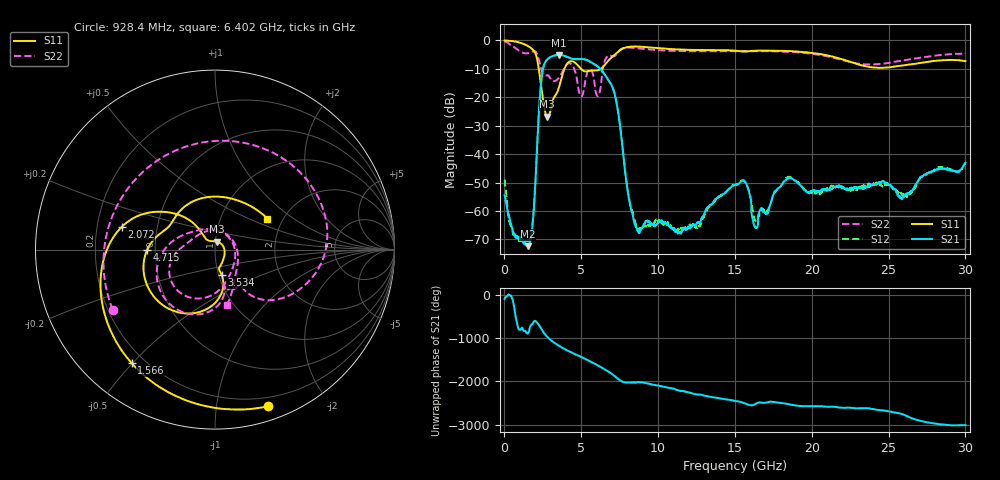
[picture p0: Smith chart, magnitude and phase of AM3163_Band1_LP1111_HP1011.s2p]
!Agilent Technologies,E8364B,MY43040894,A.07.50.67
!Agilent E8364B: A.07.50.67
!Date: Thursday, August 20, 2020 12:00:17
!Correction: S11(Full 2 Port(1,2))
!S21(Full 2 Port(1,2))
!S12(Full 2 Port(1,2))
!S22(Full 2 Port(1,2))
!S2P File: Measurements: S11, S21, S12, S22:
# Hz S  dB  R 50
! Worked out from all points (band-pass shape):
!   3201 points, 10 MHz to 30 GHz, reference 50 ohm
!   highest |S21| = -5.13 dB at 3.553 GHz (marker M1); lowest = -72.4 dB at 1.51 GHz (marker M2)
!   |S21| within 3 dB of the highest: 2.614 GHz to 5.778 GHz (3.164 GHz wide, 75.4 % of centre)
!   lowest |S11| = -26.9 dB at 2.775 GHz (marker M3), VSWR 1.09, Z = 50.7 + j4.51 ohm
!   |S11| at or under -10 dB: 2.233 GHz to 3.901 GHz (1.668 GHz wide, 54.4 % of centre); 4.978 GHz to 6.273 GHz (1.295 GHz wide, 23 % of centre)
!   |S22| runs from -19.8 to -0.3 dB; largest |S21 - S12| = 0.0055
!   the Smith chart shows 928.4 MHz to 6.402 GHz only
!   S11 on the Smith chart (normalised r, x): 928.4 MHz: 0.12, -1.39; 1.566 GHz: 0.15, -0.50; 2.072 GHz: 0.31, +0.11; 3.534 GHz: 1.03, -0.30; 4.715 GHz: 0.45, -0.00; 6.402 GHz: 1.67, +0.65
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1e7  -0.04 -4.9  -54.47 -93.1  -48.93 88.2  -0.32 -12.0
9.284438e8  -0.71 -71.3  -69.49 -77.7  -70.18 -166.5  -3.59 -149.5
1.5095e9  -1.94 -121.0  -72.36 -171.7  -70.52 24.2  -4.53 113.5
1.565731e9  -2.11 -126.4  -72.14 -146.4  -70.22 61.4  -4.47 103.4
2.071812e9  -5.44 166.3  -43.46 95.4  -43.32 96.3  -4.22 -0.9
2.774703e9  -26.89 78.8  -6.80 112.5  -6.81 112.5  -12.25 -61.4
3.140206e9  -21.27 -64.9  -5.51 0.4  -5.53 0.4  -14.26 -76.5
3.533825e9  -16.77 -75.3  -5.13 -94.0  -5.15 -94.0  -13.24 -75.8
3.552569e9  -16.45 -75.1  -5.13 -98.2  -5.15 -98.1  -13.12 -75.9
4.714681e9  -8.43 -179.4  -6.65 51.4  -6.62 51.4  -13.66 159.2
5.014581e9  -10.19 161.4  -6.55 1.0  -6.53 0.8  -19.73 33.5
6.401619e9  -9.38 30.6  -11.07 103.6  -11.14 103.5  -10.07 -77.9
7.5075e9  -3.52 -101.4  -29.36 -172.1  -29.33 -171.1  -3.41 -169.6
8.529034e9  -2.16 178.2  -65.56 129.7  -64.16 136.2  -2.72 128.7
1.000979e10  -2.76 100.6  -63.83 60.5  -63.81 -11.2  -3.45 65.6
1.227778e10  -3.36 9.7  -64.71 -124.2  -64.42 -125.2  -3.84 -15.0
1.5005e10  -3.59 -74.0  -50.86 67.0  -50.82 68.5  -3.79 -92.4
1.635455e10  -3.64 -104.2  -65.82 -0.3  -63.63 138.7  -3.79 -125.4
2.000958e10  -4.39 162.6  -52.89 -53.1  -53.58 -51.9  -4.72 135.5
2.27368e10  -7.97 60.3  -51.91 -98.3  -52.25 -102.3  -7.91 20.5
2.500479e10  -9.50 -63.1  -50.68 -172.6  -50.92 -170.0  -7.95 -93.1
3e10  -7.32 104.1  -43.03 -133.5  -43.24 -128.5  -4.65 100.5
